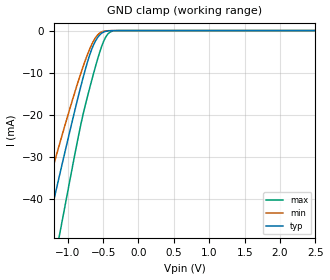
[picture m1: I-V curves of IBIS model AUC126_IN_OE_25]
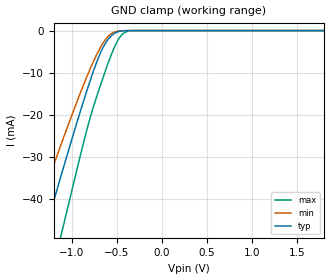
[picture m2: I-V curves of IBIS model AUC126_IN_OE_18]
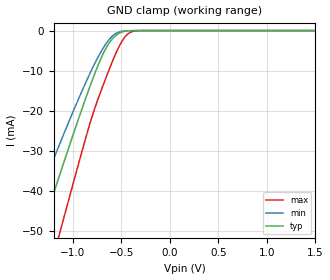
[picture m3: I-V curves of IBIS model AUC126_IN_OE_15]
| TEXAS INSTRUMENTS INCORPORATED
| Standard Linear and Logic Group
| IBIS Model of SN74AUC126
| Quadruple Bus Buffer Gate with 3-state Outputs
| This file contains package information for the following:
|  QFN 14-pin (RGY) package as [Component] AUC126_RGY
| This device can be powered at the following Vccs:
|  2.5 volt Vcc
|  1.8 volt Vcc
|  1.5 volt Vcc
|  1.2 volt Vcc
|  0.8 volt Vcc
| This file provides unique models under the [Model Selector] for each Vcc.
| For operation at a specific Vcc, select the appropriate model after each
| [Model Selector] keyword.
[IBIS Ver]   3.2
[Comment char]  |_char
[File Name]   sn74auc126.ibs
[File Rev]   1.1 | x_die
[Date]   September 15, 2003
[Source]   Data created from TI-SPICE simulations at TI-SLL.
[Notes]   The following is an IBIS list for the AUC126.
   Please contact sllibis@ti.com with questions and
   comments concerning SLL IBIS models.
   - Power clamp data deleted as there is no power-clamp diode.
   - End point warning due to AC and DC mismatch.
   - Non-monotonic data in pullup and pulldown due to
   feedback circuit.
[Disclaimer] Property of Texas Instruments Incorporated.  Unauthorized
   reproduction and/or distribution is strictly prohibited.
   This product is protected under copyright law.
   Created  2003, (C) Copyright  2003, Texas Instruments
   Incorporated, All Rights Reserved
   UNLESS THERE IS A SIGNED, WRITTEN AGREEMENT TO THE
   CONTRARY, TEXAS INSTRUMENTS (TI) IS PROVIDING THE IBIS
   MODELS  AND WITHOUT ANY WARRANTY, EXPRESSED OR
   IMPLIED.  TI assumes no liability for:
   1) the accuracy of the IBIS models provided to your
   company;
   2) the proper functioning of these IBIS Models in your
   design or for any resulting applications; or
   3) infringement of patents, copyrights or intellectual
   property rights resulting from your use of these IBIS
   models.
   TI provides IBIS Models as a service to our customers.
   You and your company shall not distribute, sell or give
   these models to anyone else without prior written
   permission from TI.
   TI reserves the right to make changes to our products or
   to discontinue any semiconductor product or service
   without notice, and advises our customers to obtain the
   latest version of relevant information to verify, before
   placing orders, that the information being relied on is
   current.
   Please be aware that your receipt and use of the IBIS
   information provided shall serve as acceptance of these
   terms and conditions.  If you do not accept these terms,
   you should return or destroy the IBIS models and any
   other accompanying information immediately.
| Component AUC126_RGY 14-pin QFN
[Component]   AUC126_RGY
[Manufacturer]   Texas Instruments, Inc.
[Package]
|   typ   min   max
R_pkg   2.900e-02   2.300e-02   4.100e-02
L_pkg   7.730e-10   6.570e-10   9.980e-10
C_pkg   1.360e-13   1.150e-13   1.560e-13
[Pin]   signal_name   model_name   R_pin   L_pin   C_pin
1   1OE   AUC126_IN_OE   2.700e-02   8.310e-10   1.300e-13
2   1A   AUC126_IN   2.700e-02   8.660e-10   1.350e-13
3   1Y   AUC126_OUT   4.100e-02   9.980e-10   1.560e-13
4   2OE   AUC126_IN_OE   3.100e-02   7.670e-10   1.420e-13
5   2A   AUC126_IN   3.100e-02   7.650e-10   1.420e-13
6   2Y   AUC126_OUT   3.100e-02   7.830e-10   1.440e-13
7   GND   GND   3.100e-02   7.810e-10   1.370e-13
8   3Y   AUC126_OUT   2.300e-02   6.570e-10   1.150e-13
9   3A   AUC126_IN   2.300e-02   8.140e-10   1.290e-13
10   3OE   AUC126_IN_OE   2.800e-02   7.040e-10   1.290e-13
11   4Y   AUC126_OUT   2.700e-02   6.720e-10   1.360e-13
12   4A   AUC126_IN   2.700e-02   6.960e-10   1.380e-13
13   4OE   AUC126_IN_OE   2.700e-02   7.250e-10   1.400e-13
14   VCC   POWER   3.000e-02   7.630e-10   1.360e-13
| Model AUC126_IN_OE
[Model Selector]   AUC126_IN_OE
AUC126_IN_OE_25   2.5 volt Vcc
AUC126_IN_OE_18   1.8 volt Vcc
AUC126_IN_OE_15   1.5 volt Vcc
AUC126_IN_OE_12   1.2 volt Vcc
AUC126_IN_OE_08   0.8 volt Vcc
| Model AUC126_IN
[Model Selector]   AUC126_IN
AUC126_IN_25   2.5 volt Vcc
AUC126_IN_18   1.8 volt Vcc
AUC126_IN_15   1.5 volt Vcc
AUC126_IN_12   1.2 volt Vcc
AUC126_IN_08   0.8 volt Vcc
| Model AUC126_OUT
[Model Selector]   AUC126_OUT
AUC126_OUT_25   2.5 volt Vcc
AUC126_OUT_18   1.8 volt Vcc
AUC126_OUT_15   1.5 volt Vcc
AUC126_OUT_12   1.2 volt Vcc
AUC126_OUT_08   0.8 volt Vcc
| Models and submodels in the file (15): AUC126_IN_OE_25 (Input), AUC126_IN_OE_18 (Input), AUC126_IN_OE_15 (Input), AUC126_IN_OE_12 (Input), AUC126_IN_OE_08 (Input), AUC126_IN_25 (Input), AUC126_IN_18 (Input), AUC126_IN_15 (Input), AUC126_IN_12 (Input), AUC126_IN_08 (Input), AUC126_OUT_25 (3-state), AUC126_OUT_18 (3-state), AUC126_OUT_15 (3-state), AUC126_OUT_12 (3-state), AUC126_OUT_08 (3-state)
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[Model]   AUC126_IN_OE_25
Model_type  Input
Vinl=0.7
Vinh=1.7
| variable   typ   min   max
C_comp   2.58pF   2.02pF   2.96pF
[Temperature Range]   40   100   -40
| Ambient temperature   25   85   -40
[Voltage range]   2.5   2.3   2.7
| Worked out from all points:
|   GND clamp passes 1 mA (typ) near -0.55 V on its own axis
[GND Clamp]
| AUC126_IN_OE_25
|   Voltage   I(typ)   I(min)   I(max)
-3.6V     -222.6mA   -186.3mA   -267.8mA
-1.485V   -61.97mA   -49.54mA   -81.7mA
-1.435V   -58.22mA   -46.44mA   -77.24mA
-1.3V     -48.12mA   -38.14mA   -65.19mA
-1.115V   -34.46mA   -27.03mA   -48.65mA
-830mV    -14.32mA   -10.98mA   -23.64mA
-720mV    -7.469mA   -5.684mA   -15.68mA
-625mV    -3.065mA   -2.183mA   -9.633mA
-525mV    -682.5uA   -363uA     -4.021mA
-430mV    -73.19uA   -35.01uA   -776.9uA
-325mV    -3.339uA   -2.017uA   -30.74uA
2.5V      328.6pA    415.9pA    485.4pA
[Model]   AUC126_IN_OE_18
Model_type  Input
Vinl=0.5775
Vinh=1.2675
| variable   typ   min   max
C_comp   2.63pF   2.14pF   3.04pF
[Temperature Range]   40   100   -40
| Ambient temperature   25   85   -40
[Voltage range]   1.8   1.65   1.95
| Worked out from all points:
|   GND clamp passes 1 mA (typ) near -0.55 V on its own axis
[GND Clamp]
| AUC126_IN_OE_18
|   Voltage   I(typ)   I(min)   I(max)
-3.6V     -222.6mA   -186.3mA   -267.8mA
-1.475V   -61.22mA   -48.92mA   -80.81mA
-1.43V    -57.84mA   -46.13mA   -76.8mA
-1.295V   -47.75mA   -37.84mA   -64.74mA
-1.1V     -33.37mA   -26.15mA   -47.31mA
-830mV    -14.32mA   -10.98mA   -23.64mA
-680mV    -5.364mA   -4.044mA   -13.09mA
-560mV    -1.272mA   -758.2uA   -5.827mA
-485mV    -290.6uA   -141.4uA   -2.305mA
-420mV    -55.81uA   -26.93uA   -608.5uA
-300mV    -1.501uA   -993.1nA   -11.88uA
1.8V      213.9pA    308.1pA    246.3pA
[Model]   AUC126_IN_OE_15
Model_type  Input
Vinl=0.49
Vinh=1.04
| variable   typ   min   max
C_comp   2.65pF   2.21pF   3.04pF
[Temperature Range]   40   100   -40
| Ambient temperature   25   85   -40
[Voltage range]   1.5   1.4   1.6
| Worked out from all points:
|   GND clamp passes 1 mA (typ) near -0.55 V on its own axis
[GND Clamp]
| AUC126_IN_OE_15
|   Voltage   I(typ)   I(min)   I(max)
-3.6V     -222.6mA   -186.3mA   -267.8mA
-1.505V   -63.48mA   -50.79mA   -83.48mA
-1.325V   -49.98mA   -39.67mA   -67.42mA
-1.17V    -38.49mA   -30.3mA    -53.57mA
-1.12V    -34.83mA   -27.33mA   -49.09mA
-840mV    -14.99mA   -11.5mA    -24.46mA
-695mV    -6.117mA   -4.635mA   -14.06mA
-570mV    -1.488mA   -916.7uA   -6.381mA
-495mV    -364.6uA   -180.3uA   -2.692mA
-430mV    -73.19uA   -35.01uA   -776.9uA
-280mV    -781.4nA   -559.2nA   -5.358uA
1.5V      174.7pA    267.7pA    181.1pA
